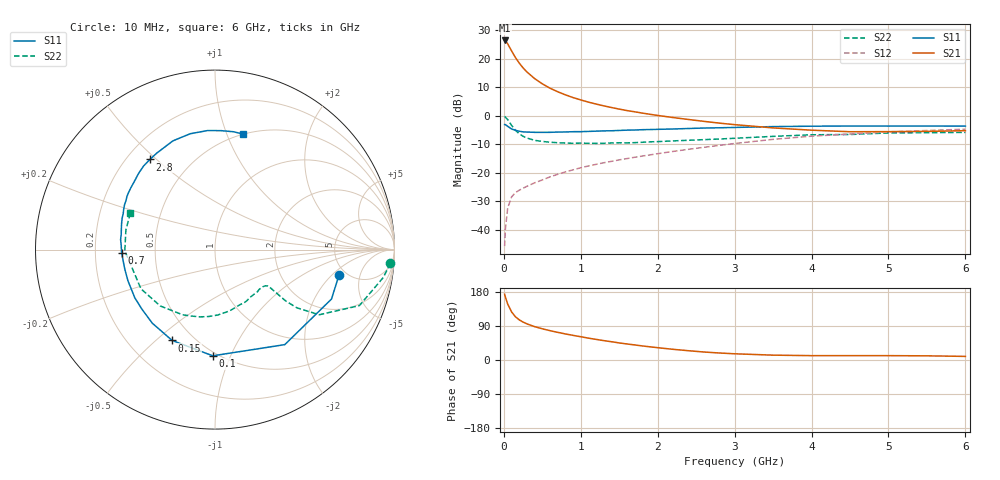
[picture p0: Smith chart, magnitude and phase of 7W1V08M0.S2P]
! Infineon Technologies  Discrete & RF Semiconductors
! BFS17W
! Si NPN RF Bipolar Junction Transistor in SOT323
! VCE = 1 V  IC = 8 mA
! Common Emitter S-Parameters:  August  1999
# GHz  S  MA  R  50
!  f  S11  S21  S12  S22
! GHz  MAG  ANG  MAG  ANG  MAG  ANG  MAG  ANG
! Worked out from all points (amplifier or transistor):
!   36 points, 10 MHz to 6 GHz, reference 50 ohm
!   highest |S21| = 26.5 dB at 10 MHz (marker M1)
!   |S21| within 3 dB of that: start of sweep to 87.15 MHz
!   unconditionally stable (mu >= 1): 385.1 MHz to end of sweep
!   at 250 MHz: K = 0.78, MSG = 21.1 dB, |S12| = -25.4 dB
!   at 1.4 GHz: K = 1.31, MAG = 6.1 dB, |S12| = -15.9 dB
!   at 6 GHz: K = 1.12, MAG = -2.3 dB, |S12| = -4.7 dB
!   S11 on the Smith chart (normalised r, x): 10 MHz: 4.37, -2.45; 100 MHz: 0.47, -0.86; 150 MHz: 0.38, -0.56; 700 MHz: 0.32, -0.01; 2.8 GHz: 0.29, +0.48; 6 GHz: 0.50, +1.15
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0.01  0.7056 -11.5  21.04 173.6  0.0052 83.6  0.9804 -4.4
0.02  0.7051 -23.0  20.71 166.2  0.0104 82.2  0.9505 -9.4
0.05  0.6569 -53.7  18.38 147.8  0.0242 66.2  0.863 -21.2
0.1  0.5919 -91.2  13.85 127.1  0.0379 53.4  0.6849 -32.0
0.15  0.5597 -115.3  10.6 114.2  0.0451 47.9  0.5604 -35.4
0.2  0.5386 -130.5  8.443 106.0  0.0498 47.1  0.487 -36.0
0.25  0.5251 -141.1  6.953 100.0  0.0539 46.9  0.4388 -35.5
0.3  0.5213 -149.0  5.897 95.4  0.0583 48.6  0.4104 -35.1
0.4  0.5153 -160.2  4.513 88.0  0.0671 50.7  0.3733 -34.6
0.5  0.5143 -167.9  3.653 82.4  0.0754 53.5  0.357 -34.6
0.6  0.5157 -173.4  3.063 77.4  0.0853 55.0  0.3461 -35.6
0.7  0.5208 -178.2  2.655 73.0  0.0946 56.4  0.3388 -37.4
0.9  0.529 173.9  2.095 65.0  0.1133 58.3  0.331 -42.2
1.1  0.5351 167.1  1.744 57.7  0.1325 59.0  0.331 -48.0
1.3  0.5465 161.1  1.5 51.1  0.151 59.3  0.3306 -54.9
1.6  0.5629 153.5  1.241 42.3  0.1785 59.3  0.3368 -65.3
2.2  0.5895 139.3  0.936 28.2  0.2385 58.4  0.3646 -87.5
2.8  0.6194 125.8  0.748 18.5  0.3041 55.4  0.3932 -109.7
3.5  0.6496 111.2  0.616 12.8  0.388 49.3  0.4379 -134.2
4.5  0.6646 93.5  0.528 11.5  0.4805 37.2  0.4724 -167.0
5.5  0.6647 81.0  0.535 11.0  0.5551 26.2  0.5084 167.6
6  0.6623 76.2  0.551 9.5  0.585 20.9  0.5137 156.5
